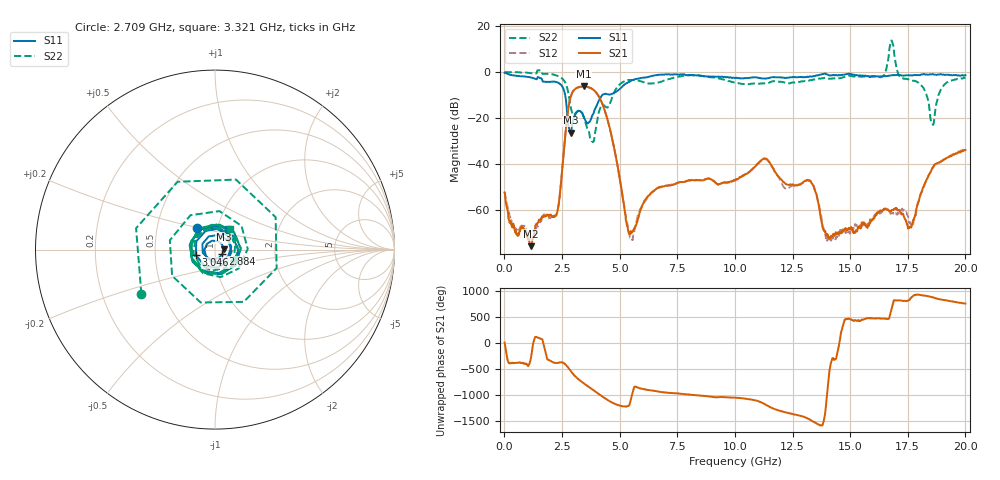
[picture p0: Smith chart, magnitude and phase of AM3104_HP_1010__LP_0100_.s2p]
!Created with skrf (http://scikit-rf.org).
# Hz S RI R 50.0
!freq ReS11 ImS11 ReS21 ImS21 ReS12 ImS12 ReS22 ImS22
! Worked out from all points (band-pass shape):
!   1601 points, 10 MHz to 20 GHz, reference 50 ohm
!   highest |S21| = -6.28 dB at 3.433 GHz (marker M1); lowest = -75.5 dB at 1.147 GHz (marker M2)
!   |S21| within 3 dB of the highest: 2.93 GHz to 4.012 GHz (1.082 GHz wide, 31.2 % of centre)
!   lowest |S11| = -26.3 dB at 2.871 GHz (marker M3), VSWR 1.10, Z = 55.1 + j0.259 ohm
!   |S11| at or under -10 dB: 2.637 GHz to 4.249 GHz (1.612 GHz wide, 46.8 % of centre)
!   |S22| runs from -30.4 to 13.7 dB; largest |S21 - S12| = 0.022
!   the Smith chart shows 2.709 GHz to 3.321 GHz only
!   S11 on the Smith chart (normalised r, x): 2.709 GHz: 0.80, +0.19; 2.884 GHz: 1.09, -0.05; 3.046 GHz: 0.81, -0.05; 3.321 GHz: 1.12, +0.26
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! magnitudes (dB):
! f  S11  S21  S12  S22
! 10 MHz  -0.3  -52.3  -51.9  -0.1
! 1.147 GHz  -2.4  -75.5  -72.7  -0.5
! 2.271 GHz  -4.4  -61.3  -61.6  -1.6
! 2.709 GHz  -16.3  -20.9  -20.9  -6.4
! 2.871 GHz  -26.3  -11.0  -11.0  -14.8
! 2.884 GHz  -26.3  -10.5  -10.6  -15.5
! 3.046 GHz  -19.1  -7.6  -7.6  -18.2
! 3.321 GHz  -17.3  -6.4  -6.5  -17.0
! 3.346 GHz  -17.5  -6.4  -6.4  -17.2
! 3.433 GHz  -19.2  -6.3  -6.3  -19.4
! 3.808 GHz  -19.0  -7.3  -7.4  -30.2
! 4.383 GHz  -9.5  -17.6  -17.7  -15.1
! 5.47 GHz  -4.0  -70.3  -72.7  -3.5
! 6.682 GHz  -1.2  -50.1  -50.2  -4.6
! 10.01 GHz  -2.7  -47.0  -47.2  -4.6
! 11.3 GHz  -2.9  -37.6  -37.8  -5.0
! 13.34 GHz  -2.0  -48.4  -48.0  -3.5
! 14.08 GHz  -1.5  -71.6  -73.0  -2.9
! 16.68 GHz  -1.6  -60.0  -60.7  7.2
! 17.6 GHz  -1.5  -67.3  -65.2  -3.5
! 18.56 GHz  -0.9  -41.7  -41.9  -22.6
! 20 GHz  -1.4  -33.8  -33.4  -2.5
